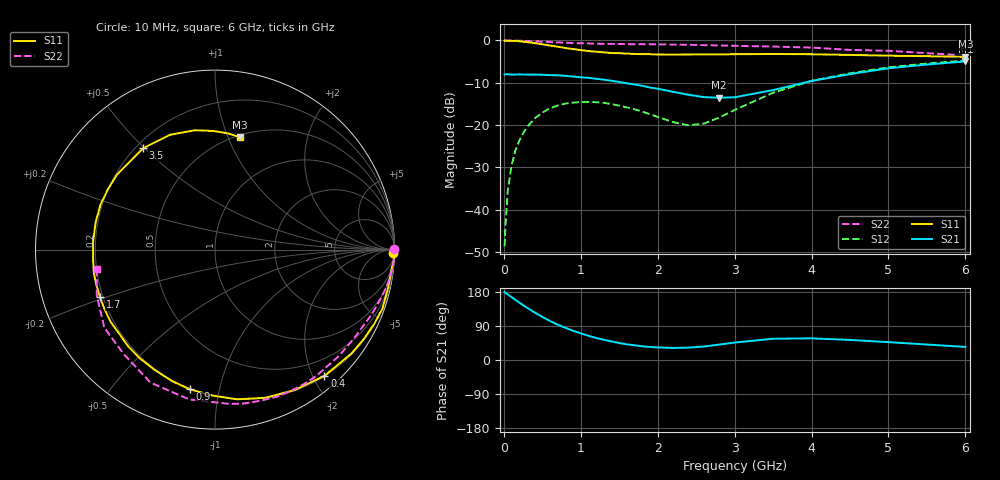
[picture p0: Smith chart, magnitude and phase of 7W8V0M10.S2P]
! Infineon Technologies  Discrete & RF Semiconductors
! BFS17W
! Si NPN RF Bipolar Junction Transistor in SOT323
! VCE = 8 V  IC = 0.1 mA
! Common Emitter S-Parameters:  August  1999
# GHz  S  MA  R  50
!  f  S11  S21  S12  S22
! GHz  MAG  ANG  MAG  ANG  MAG  ANG  MAG  ANG
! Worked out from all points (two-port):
!   36 points, 10 MHz to 6 GHz, reference 50 ohm
!   highest |S21| = -4.96 dB at 6 GHz (marker M1); lowest = -13.6 dB at 2.8 GHz (marker M2)
!   |S21| within 3 dB of the highest: 4.5 GHz to end of sweep
!   lowest |S11| = -3.9 dB at 6 GHz (marker M3), VSWR 4.56, Z = 26 + j55.1 ohm
!   |S11| at or under -10 dB: nowhere
!   |S22| runs from -3.5 to 0.0 dB; largest |S21 - S12| = 0.4
!   S11 on the Smith chart (normalised r, x): 10 MHz: open; 400 MHz: 0.21, -2.17; 900 MHz: 0.20, -0.82; 1.7 GHz: 0.19, -0.19; 3.5 GHz: 0.23, +0.49; 6 GHz: 0.52, +1.10
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0.01  0.9939 -1.1  0.396 179.5  0.0037 89.0  0.9999 0.1
0.02  0.9999 -2.8  0.399 177.3  0.0061 91.5  0.9918 -0.6
0.05  0.9892 -6.3  0.399 173.0  0.0165 87.8  0.9985 -1.7
0.1  0.9875 -12.3  0.395 166.1  0.0332 82.5  0.9997 -3.3
0.15  0.9892 -19.4  0.395 158.7  0.0499 77.4  0.9953 -4.9
0.2  0.9787 -25.1  0.397 151.7  0.0652 74.7  0.9921 -6.5
0.3  0.9555 -37.4  0.395 138.2  0.0943 66.6  0.9853 -9.6
0.4  0.9309 -49.1  0.395 125.3  0.1195 59.3  0.9761 -12.7
0.6  0.8718 -71.3  0.389 102.9  0.1578 46.4  0.9569 -18.2
0.9  0.791 -100.2  0.374 76.9  0.1841 31.1  0.9318 -26.2
1.1  0.7495 -116.8  0.362 63.9  0.1881 23.3  0.9211 -31.3
1.3  0.724 -132.0  0.344 53.5  0.1834 17.2  0.9123 -36.5
1.7  0.6928 -157.7  0.302 38.8  0.1534 10.9  0.9015 -47.2
2.2  0.6806 176.2  0.247 31.8  0.1084 21.9  0.8944 -61.2
2.4  0.6822 167.0  0.228 32.7  0.0992 35.1  0.8891 -67.2
2.8  0.6848 150.2  0.21 40.7  0.1225 63.1  0.873 -79.1
3.5  0.6922 125.4  0.259 56.1  0.241 73.7  0.8471 -99.7
4  0.6868 111.3  0.332 57.1  0.3332 67.6  0.8236 -115.8
4.5  0.6744 99.5  0.4 53.0  0.4089 59.5  0.7732 -131.1
5  0.6609 90.7  0.469 47.1  0.4813 51.5  0.7549 -144.7
5.5  0.6514 83.2  0.519 40.8  0.5334 43.6  0.7068 -158.8
6  0.6403 77.6  0.565 34.5  0.5786 36.5  0.6667 -170.9
